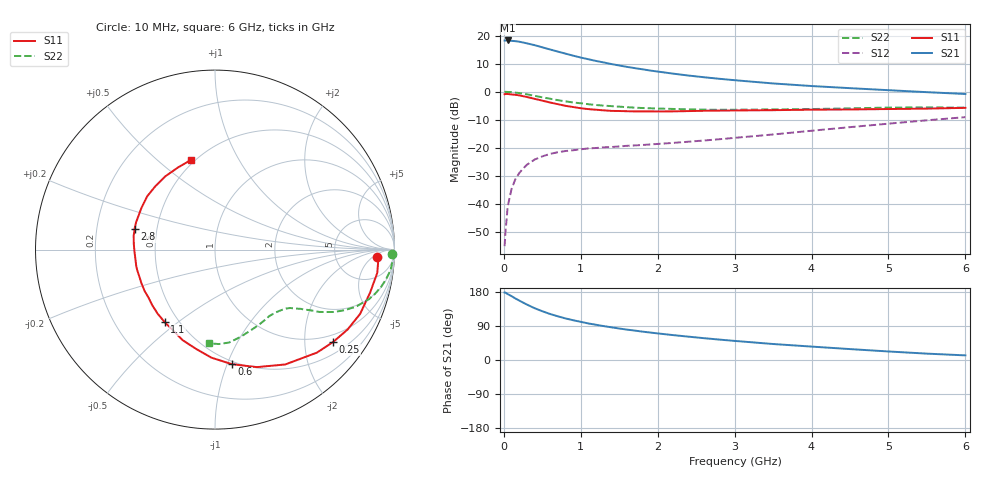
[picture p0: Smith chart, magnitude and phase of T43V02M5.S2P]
! Infineon Technologies  Discrete & RF Semiconductors
! BFR182T
! Si NPN RF Bipolar Junction Transistor in SC75
! VCE = 3 V  IC = 2.5 mA
! Common Emitter S-Parameters:  October  1999
# GHz  S  MA  R  50
!  f  S11  S21  S12  S22
! GHz  MAG  ANG  MAG  ANG  MAG  ANG  MAG  ANG
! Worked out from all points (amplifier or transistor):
!   36 points, 10 MHz to 6 GHz, reference 50 ohm
!   highest |S21| = 18.2 dB at 50 MHz (marker M1)
!   |S21| within 3 dB of that: start of sweep to 573.9 MHz
!   unconditionally stable (mu >= 1): 1.841 GHz to 4.25 GHz
!   at 250 MHz: K = 0.17, MSG = 22.4 dB, |S12| = -27.3 dB
!   at 1.4 GHz: K = 0.84, MSG = 14.7 dB, |S12| = -19.6 dB
!   at 6 GHz: K = 0.83, MSG = 4.1 dB, |S12| = -9.0 dB
!   lowest NFmin = 1.10 dB at 450 MHz
!   S11 on the Smith chart (normalised r, x): 10 MHz: 16, -7; 250 MHz: 0.79, -2.70; 600 MHz: 0.48, -1.04; 1.1 GHz: 0.42, -0.45; 2.8 GHz: 0.37, +0.11; 6 GHz: 0.48, +0.65
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0.01  0.903 -2.6  8.139 178.2  0.0018 89.0  0.9883 -1.4
0.02  0.9126 -2.0  8.136 177.9  0.003 92.4  0.9984 -1.4
0.05  0.9133 -8.2  8.17 174.0  0.0091 88.7  0.9918 -3.4
0.1  0.8965 -15.6  8.056 168.5  0.0187 83.6  0.9849 -6.6
0.15  0.8843 -23.9  7.935 162.4  0.028 76.3  0.9673 -9.8
0.25  0.8356 -38.0  7.519 151.5  0.043 69.6  0.9254 -15.4
0.3  0.8075 -45.3  7.256 146.3  0.0505 66.7  0.9019 -17.8
0.4  0.7499 -58.6  6.74 136.7  0.0624 60.3  0.8481 -22.0
0.5  0.695 -70.4  6.171 128.7  0.071 55.9  0.7978 -25.0
0.6  0.6452 -81.6  5.653 121.5  0.0786 51.8  0.7525 -27.5
0.7  0.6024 -91.9  5.187 115.4  0.0841 49.5  0.7107 -29.3
0.8  0.5632 -100.8  4.772 109.8  0.0884 47.3  0.6761 -30.9
0.9  0.5357 -109.7  4.388 105.0  0.0913 46.0  0.6457 -31.9
1.1  0.4915 -124.9  3.784 96.4  0.0985 43.9  0.6009 -33.8
1.3  0.4672 -138.5  3.318 89.4  0.103 43.8  0.5669 -35.5
1.6  0.4509 -155.2  2.771 80.2  0.1095 44.4  0.532 -37.7
2.2  0.4485 -178.2  2.101 65.7  0.1234 48.7  0.4953 -43.5
2.8  0.4629 165.5  1.702 53.9  0.1432 53.3  0.4779 -50.9
3.5  0.4709 150.7  1.406 42.2  0.1742 57.4  0.4852 -59.8
4.5  0.4848 133.3  1.159 28.8  0.235 58.9  0.5073 -74.1
5.5  0.5021 114.1  0.984 16.8  0.3112 56.1  0.5268 -87.7
6  0.5176 104.8  0.913 12.2  0.354 53.0  0.5227 -93.8
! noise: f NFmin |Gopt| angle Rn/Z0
0.45  1.1  0.39  29  0.35
0.9  1.2  0.37  59  0.28
1.8  1.8  0.28  128  0.2
